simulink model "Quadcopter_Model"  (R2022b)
settings: Solver=VariableStepAuto  StartTime=0.0  StopTime=runtime  FixedStep=0.001  RelTol=1e-3
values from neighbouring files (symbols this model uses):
  delta_T = [ 0,  0,  9.404e-04 ]    [modelParameters.m]    (also in rich_params.m = [ 0,  0,  1.176e-04 ]; drone_control_system_test.m)
  g = 9.81    [modelParameters.m]    (also in rich_params.m; drone_control_system_test.m; imu_model_test.m = 0.1)
  height_controlled_o = (((Rm*If        + (((omega0_o * 2 * Rm * Kv * Kq      * Kd + 1)^2) - 1)/(4* Rm*Kv^2*Kq      * Kd))/Vb)*(Pmax - Pmin) + Pmin)    [modelParameters.m]    (also in rich_params.m)
  If = 0.3836    [modelParameters.m]    (also in rich_params.m = 0.39; drone_control_system_test.m)
  Jreq = 4.2012e-05    [modelParameters.m]    (also in rich_params.m = 1.376e-05; drone_control_system_test.m)
  Jxx = 0.0110    (= 0.011)    [modelParameters.m]    (also in rich_params.m = 0.0081; drone_control_system_test.m)
  Jyy = 0.0116    [modelParameters.m]    (also in rich_params.m = 0.0074; drone_control_system_test.m)
  Jzz = 0.0223    [modelParameters.m]    (also in rich_params.m = 0.0135; drone_control_system_test.m)
  Kd = 1.4852e-07    [modelParameters.m]    (also in rich_params.m = 5.194e-07; drone_control_system_test.m)
  Kh = 3.4574e-04    (= 0.00034574)    [modelParameters.m]    (also in rich_params.m; drone_control_system_test.m)
  Kq = 96.3422    [modelParameters.m]    (also in rich_params.m = 110; drone_control_system_test.m)
  Kt = 1.2007e-05    [modelParameters.m]    (also in rich_params.m = 7.3956e-06; drone_control_system_test.m)
  Kv = 96.3422    [modelParameters.m]    (also in rich_params.m = 110; drone_control_system_test.m)
  m = 1.216    [modelParameters.m]    (also in rich_params.m = 0.656; drone_control_system_test.m)
  omega0_o = sqrt((m*g)/(4*Kt))    [modelParameters.m]    (also in rich_params.m)
  omega1_o = sqrt((m*g)/(4*Kt))    [modelParameters.m]    (also in rich_params.m)
  omega2_o = sqrt((m*g)/(4*Kt))    [modelParameters.m]    (also in rich_params.m)
  omega3_o = sqrt((m*g)/(4*Kt))    [modelParameters.m]    (also in rich_params.m)
  pitch_o = 0    [modelParameters.m]    (also in rich_params.m)
  pitchrate_o = 0    [modelParameters.m]    (also in rich_params.m)
  Pmax = 1    [modelParameters.m]    (also in rich_params.m; drone_control_system_test.m)
  Pmin = 0    [modelParameters.m]    (also in rich_params.m; drone_control_system_test.m)
  r_oc = [ 0 ; 0 ; 0 ]    [modelParameters.m]    (also in rich_params.m; drone_control_system_test.m = [0; 0; 0]; imu_model_test.m = 0.1)
  rhx = 0.16    [modelParameters.m]    (also in rich_params.m = 0.115; drone_control_system_test.m)
  rhy = 0.16    [modelParameters.m]    (also in rich_params.m = 0.115; drone_control_system_test.m)
  rhz = 0.03    [modelParameters.m]    (also in rich_params.m = 0.04; drone_control_system_test.m)
  Rm = 0.235    [modelParameters.m]    (also in rich_params.m = 0.19; drone_control_system_test.m)
  roll_o = 0    [modelParameters.m]    (also in rich_params.m)
  rollrate_o = 0    [modelParameters.m]    (also in rich_params.m)
  signal_mixer = [ 1, -1, -1, -1    [modelParameters.m]    (also in rich_params.m; drone_control_system_test.m)
  Tc = 0.01    [modelParameters.m]    (also in rich_params.m; drone_control_system_test.m)
  Tq = 0.005    [modelParameters.m]    (also in rich_params.m; drone_control_system_test.m)
  Vb = 12.3    [modelParameters.m]    (also in rich_params.m = 11.4; drone_control_system_test.m)
  x_controlled_o = 0    [modelParameters.m]    (also in rich_params.m)
  x_o = 0    [modelParameters.m]    (also in rich_params.m)
  x_vel_o = 0    [modelParameters.m]    (also in rich_params.m)
  y_controlled_o = 0    [modelParameters.m]    (also in rich_params.m)
  y_o = 0    [modelParameters.m]    (also in rich_params.m)
  y_vel_o = 0    [modelParameters.m]    (also in rich_params.m)
  yaw_controlled_o = 0    [modelParameters.m]    (also in rich_params.m)
  yaw_o = 0    [modelParameters.m]    (also in rich_params.m)
  yawrate_o = 0    [modelParameters.m]    (also in rich_params.m)
  z_o = 0    [modelParameters.m]    (also in rich_params.m)
  z_vel_o = 0    [modelParameters.m]    (also in rich_params.m)
undefined symbols (not defined in the file or in its folder): lqr_K
libraries: Derivative x13, slpidlib x13, dsparch4 x3, vrlib x2, simulink_need_slupdate x2, simulink x1
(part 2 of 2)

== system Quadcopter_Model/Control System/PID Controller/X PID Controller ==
  x_error : Inport
  x_pos : Inport  Port=2
  Add : Sum  Inputs=+-
  Discrete D Controller : Derivative/Discrete D Controller  Kd=Kd  a=a
  Discrete PI Controller : slpidlib/PID Controller  Controller=PI  Form=Parallel  TimeDomain=Discrete-time  UseExternalTs=off  SampleTime=Ts  IntegratorMethod=Forward Euler  FilterMethod=Forward Euler  ControllerParametersSource=internal  P=Kp  I=Ki  UseKiTs=off  D=0  N=100  UseFilter=on  TunerSelectOption=Transfer Function Based (PID Tuner App)  InitialConditionSource=internal  InitialConditionForIntegrator=0  InitialConditionForFilter=0  DifferentiatorICPrevScaledInput=0  ExternalReset=none  TrackingMode=off  Kt=1  LimitOutput=off  SatLimitsSource=internal  UpperSaturationLimit=inf  LowerSaturationLimit=-inf  LinearizeAsGain=off  AntiWindupMode=none  Kb=1  LimitIntegrator=off  UpperIntegratorSaturationLimit=inf  LowerIntegratorSaturationLimit=-inf  POutMin=[]  POutMax=[]  IOutMin=[]  IOutMax=[]  DOutMin=[]  DOutMax=[]  NOutMin=[]  NOutMax=[]  SumOutMin=[]  SumOutMax=[]  SaturationOutMin=[]  SaturationOutMax=[]  PParamMin=[]  PParamMax=[]  IParamMin=[]  IParamMax=[]  DParamMin=[]  DParamMax=[]  NParamMin=[]  NParamMax=[]  KbParamMin=[]  KbParamMax=[]  KtParamMin=[]  KtParamMax=[]  KbOutMin=[]  KbOutMax=[]  KtOutMin=[]  KtOutMax=[]  IntegratorOutMin=[]  IntegratorOutMax=[]  FilterOutMin=[]  FilterOutMax=[]  SumI1OutMin=[]  SumI1OutMax=[]  SumI2OutMin=[]  SumI2OutMax=[]  SumI3OutMin=[]  SumI3OutMax=[]  SumI4OutMin=[]  SumI4OutMax=[]  SumDOutMin=[]  SumDOutMax=[]  DifferentiatorOutMin=[]  DifferentiatorOutMax=[]  FilterDiffOutCoefMin=[]  FilterDiffOutCoefMax=[]  ReciprocalOutMin=[]  ReciprocalOutMax=[]  SumDenOutMin=[]  SumDenOutMax=[]  SumNumOutMin=[]  SumNumOutMax=[]  DivideOutMin=[]  DivideOutMax=[]  UdiffTsProdOutMin=[]  UdiffTsProdOutMax=[]  NTsProdOutMin=[]  NTsProdOutMax=[]  UintegralTsProdOutMin=[]  UintegralTsProdOutMax=[]  UngainTsProdOutMin=[]  UngainTsProdOutMax=[]  ClampingZeroOutDataTypeStr=Inherit: Inherit via back propagation  ClampingZeroOutMin=[]  ClampingZeroOutMax=[]  FilterDenConstantOutDataTypeStr=Inherit: Inherit via back propagation  FilterDenConstantOutMin=[]  FilterDenConstantOutMax=[]  PCopyOutDataTypeStr=Inherit: Inherit via back propagation  PCopyOutMin=[]  PCopyOutMax=[]  NCopyOutDataTypeStr=Inherit: Inherit via back propagation  NCopyOutMin=[]  NCopyOutMax=[]  IntegratorContinuousStateAttributes=''  IntegratorStateMustResolveToSignalObject=off  IntegratorRTWStateStorageClass=Auto  FilterContinuousStateAttributes=''  FilterStateMustResolveToSignalObject=off  FilterRTWStateStorageClass=Auto  ParallelPVariant=InternalParameters  IdealPVariant=Disabled  IVariant=InternalParameters  DVariant=Disabled  IntegratorVariant=Discrete  SatVariant=Disabled  AWVariant=Passthrough  PCopyVariant=Disabled  TRVariant=Disabled  FdbkBlocksVariant=Forward  IdealPFdbkVariant=Disabled  SatFdbkVariant=Disabled  DerivativeFilterVariant=Disabled  NVariant=Disabled  NCopyVariant=Disabled_SignalSpec  FilterICVariant=Disabled  IntegratorICVariant=InternalICs  ExternalResetVariant=Disabled  TRSumVariant=Passthrough  SumFdbkVariant=Disabled  SumVariant=Sum_PI  TsampFilterVariant=InternalTs  TsampNgainVariant=Passthrough  TsampIntegralVariant=Passthrough  ExternalSaturationOutDataTypeStr=Inherit: Same as second input
  pitch_setpoint : Outport
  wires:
  x_pos/1 -> Discrete D Controller/1
  x_error/1 -> Discrete PI Controller/1
  Discrete PI Controller/1 -> Add/1
  Discrete D Controller/1 -> Add/2
  Add/1 -> pitch_setpoint/1

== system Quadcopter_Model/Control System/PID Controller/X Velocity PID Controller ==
  x_vel_error : Inport
  x_vel : Inport  Port=2
  Add : Sum  Inputs=+-
  Discrete D Controller : Derivative/Discrete D Controller  Kd=Kd  a=a
  Discrete PI Controller : slpidlib/PID Controller  Controller=PI  Form=Parallel  TimeDomain=Discrete-time  UseExternalTs=off  SampleTime=Ts  IntegratorMethod=Forward Euler  FilterMethod=Forward Euler  ControllerParametersSource=internal  P=Kp  I=Ki  UseKiTs=off  D=0  N=100  UseFilter=on  TunerSelectOption=Transfer Function Based (PID Tuner App)  InitialConditionSource=internal  InitialConditionForIntegrator=0  InitialConditionForFilter=0  DifferentiatorICPrevScaledInput=0  ExternalReset=none  TrackingMode=off  Kt=1  LimitOutput=off  SatLimitsSource=internal  UpperSaturationLimit=inf  LowerSaturationLimit=-inf  LinearizeAsGain=off  AntiWindupMode=none  Kb=1  LimitIntegrator=off  UpperIntegratorSaturationLimit=inf  LowerIntegratorSaturationLimit=-inf  POutMin=[]  POutMax=[]  IOutMin=[]  IOutMax=[]  DOutMin=[]  DOutMax=[]  NOutMin=[]  NOutMax=[]  SumOutMin=[]  SumOutMax=[]  SaturationOutMin=[]  SaturationOutMax=[]  PParamMin=[]  PParamMax=[]  IParamMin=[]  IParamMax=[]  DParamMin=[]  DParamMax=[]  NParamMin=[]  NParamMax=[]  KbParamMin=[]  KbParamMax=[]  KtParamMin=[]  KtParamMax=[]  KbOutMin=[]  KbOutMax=[]  KtOutMin=[]  KtOutMax=[]  IntegratorOutMin=[]  IntegratorOutMax=[]  FilterOutMin=[]  FilterOutMax=[]  SumI1OutMin=[]  SumI1OutMax=[]  SumI2OutMin=[]  SumI2OutMax=[]  SumI3OutMin=[]  SumI3OutMax=[]  SumI4OutMin=[]  SumI4OutMax=[]  SumDOutMin=[]  SumDOutMax=[]  DifferentiatorOutMin=[]  DifferentiatorOutMax=[]  FilterDiffOutCoefMin=[]  FilterDiffOutCoefMax=[]  ReciprocalOutMin=[]  ReciprocalOutMax=[]  SumDenOutMin=[]  SumDenOutMax=[]  SumNumOutMin=[]  SumNumOutMax=[]  DivideOutMin=[]  DivideOutMax=[]  UdiffTsProdOutMin=[]  UdiffTsProdOutMax=[]  NTsProdOutMin=[]  NTsProdOutMax=[]  UintegralTsProdOutMin=[]  UintegralTsProdOutMax=[]  UngainTsProdOutMin=[]  UngainTsProdOutMax=[]  ClampingZeroOutDataTypeStr=Inherit: Inherit via back propagation  ClampingZeroOutMin=[]  ClampingZeroOutMax=[]  FilterDenConstantOutDataTypeStr=Inherit: Inherit via back propagation  FilterDenConstantOutMin=[]  FilterDenConstantOutMax=[]  PCopyOutDataTypeStr=Inherit: Inherit via back propagation  PCopyOutMin=[]  PCopyOutMax=[]  NCopyOutDataTypeStr=Inherit: Inherit via back propagation  NCopyOutMin=[]  NCopyOutMax=[]  IntegratorContinuousStateAttributes=''  IntegratorStateMustResolveToSignalObject=off  IntegratorRTWStateStorageClass=Auto  FilterContinuousStateAttributes=''  FilterStateMustResolveToSignalObject=off  FilterRTWStateStorageClass=Auto  ParallelPVariant=InternalParameters  IdealPVariant=Disabled  IVariant=InternalParameters  DVariant=Disabled  IntegratorVariant=Discrete  SatVariant=Disabled  AWVariant=Passthrough  PCopyVariant=Disabled  TRVariant=Disabled  FdbkBlocksVariant=Forward  IdealPFdbkVariant=Disabled  SatFdbkVariant=Disabled  DerivativeFilterVariant=Disabled  NVariant=Disabled  NCopyVariant=Disabled_SignalSpec  FilterICVariant=Disabled  IntegratorICVariant=InternalICs  ExternalResetVariant=Disabled  TRSumVariant=Passthrough  SumFdbkVariant=Disabled  SumVariant=Sum_PI  TsampFilterVariant=InternalTs  TsampNgainVariant=Passthrough  TsampIntegralVariant=Passthrough  ExternalSaturationOutDataTypeStr=Inherit: Same as second input
  pitch_setpoint : Outport
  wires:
  x_vel/1 -> Discrete D Controller/1
  x_vel_error/1 -> Discrete PI Controller/1
  Discrete PI Controller/1 -> Add/1
  Discrete D Controller/1 -> Add/2
  Add/1 -> pitch_setpoint/1

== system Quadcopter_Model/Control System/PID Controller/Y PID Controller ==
  y_error : Inport
  y_pos : Inport  Port=2
  Add : Sum  Inputs=+-
  Discrete D Controller : Derivative/Discrete D Controller  Kd=Kd  a=a
  Discrete PI Controller : slpidlib/PID Controller  Controller=PI  Form=Parallel  TimeDomain=Discrete-time  UseExternalTs=off  SampleTime=Ts  IntegratorMethod=Forward Euler  FilterMethod=Forward Euler  ControllerParametersSource=internal  P=Kp  I=Ki  UseKiTs=off  D=0  N=100  UseFilter=on  TunerSelectOption=Transfer Function Based (PID Tuner App)  InitialConditionSource=internal  InitialConditionForIntegrator=0  InitialConditionForFilter=0  DifferentiatorICPrevScaledInput=0  ExternalReset=none  TrackingMode=off  Kt=1  LimitOutput=off  SatLimitsSource=internal  UpperSaturationLimit=inf  LowerSaturationLimit=-inf  LinearizeAsGain=off  AntiWindupMode=none  Kb=1  LimitIntegrator=off  UpperIntegratorSaturationLimit=inf  LowerIntegratorSaturationLimit=-inf  POutMin=[]  POutMax=[]  IOutMin=[]  IOutMax=[]  DOutMin=[]  DOutMax=[]  NOutMin=[]  NOutMax=[]  SumOutMin=[]  SumOutMax=[]  SaturationOutMin=[]  SaturationOutMax=[]  PParamMin=[]  PParamMax=[]  IParamMin=[]  IParamMax=[]  DParamMin=[]  DParamMax=[]  NParamMin=[]  NParamMax=[]  KbParamMin=[]  KbParamMax=[]  KtParamMin=[]  KtParamMax=[]  KbOutMin=[]  KbOutMax=[]  KtOutMin=[]  KtOutMax=[]  IntegratorOutMin=[]  IntegratorOutMax=[]  FilterOutMin=[]  FilterOutMax=[]  SumI1OutMin=[]  SumI1OutMax=[]  SumI2OutMin=[]  SumI2OutMax=[]  SumI3OutMin=[]  SumI3OutMax=[]  SumI4OutMin=[]  SumI4OutMax=[]  SumDOutMin=[]  SumDOutMax=[]  DifferentiatorOutMin=[]  DifferentiatorOutMax=[]  FilterDiffOutCoefMin=[]  FilterDiffOutCoefMax=[]  ReciprocalOutMin=[]  ReciprocalOutMax=[]  SumDenOutMin=[]  SumDenOutMax=[]  SumNumOutMin=[]  SumNumOutMax=[]  DivideOutMin=[]  DivideOutMax=[]  UdiffTsProdOutMin=[]  UdiffTsProdOutMax=[]  NTsProdOutMin=[]  NTsProdOutMax=[]  UintegralTsProdOutMin=[]  UintegralTsProdOutMax=[]  UngainTsProdOutMin=[]  UngainTsProdOutMax=[]  ClampingZeroOutDataTypeStr=Inherit: Inherit via back propagation  ClampingZeroOutMin=[]  ClampingZeroOutMax=[]  FilterDenConstantOutDataTypeStr=Inherit: Inherit via back propagation  FilterDenConstantOutMin=[]  FilterDenConstantOutMax=[]  PCopyOutDataTypeStr=Inherit: Inherit via back propagation  PCopyOutMin=[]  PCopyOutMax=[]  NCopyOutDataTypeStr=Inherit: Inherit via back propagation  NCopyOutMin=[]  NCopyOutMax=[]  IntegratorContinuousStateAttributes=''  IntegratorStateMustResolveToSignalObject=off  IntegratorRTWStateStorageClass=Auto  FilterContinuousStateAttributes=''  FilterStateMustResolveToSignalObject=off  FilterRTWStateStorageClass=Auto  ParallelPVariant=InternalParameters  IdealPVariant=Disabled  IVariant=InternalParameters  DVariant=Disabled  IntegratorVariant=Discrete  SatVariant=Disabled  AWVariant=Passthrough  PCopyVariant=Disabled  TRVariant=Disabled  FdbkBlocksVariant=Forward  IdealPFdbkVariant=Disabled  SatFdbkVariant=Disabled  DerivativeFilterVariant=Disabled  NVariant=Disabled  NCopyVariant=Disabled_SignalSpec  FilterICVariant=Disabled  IntegratorICVariant=InternalICs  ExternalResetVariant=Disabled  TRSumVariant=Passthrough  SumFdbkVariant=Disabled  SumVariant=Sum_PI  TsampFilterVariant=InternalTs  TsampNgainVariant=Passthrough  TsampIntegralVariant=Passthrough  ExternalSaturationOutDataTypeStr=Inherit: Same as second input
  roll_setpoint : Outport
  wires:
  y_pos/1 -> Discrete D Controller/1
  y_error/1 -> Discrete PI Controller/1
  Discrete PI Controller/1 -> Add/1
  Discrete D Controller/1 -> Add/2
  Add/1 -> roll_setpoint/1

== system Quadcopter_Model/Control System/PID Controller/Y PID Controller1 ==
  y_error : Inport
  y_pos : Inport  Port=2
  Add : Sum  Inputs=+-
  Discrete D Controller : Derivative/Discrete D Controller  Kd=Kd  a=a
  Discrete PI Controller : slpidlib/PID Controller  Controller=PI  Form=Parallel  TimeDomain=Discrete-time  UseExternalTs=off  SampleTime=Ts  IntegratorMethod=Forward Euler  FilterMethod=Forward Euler  ControllerParametersSource=internal  P=Kp  I=Ki  UseKiTs=off  D=0  N=100  UseFilter=on  TunerSelectOption=Transfer Function Based (PID Tuner App)  InitialConditionSource=internal  InitialConditionForIntegrator=0  InitialConditionForFilter=0  DifferentiatorICPrevScaledInput=0  ExternalReset=none  TrackingMode=off  Kt=1  LimitOutput=off  SatLimitsSource=internal  UpperSaturationLimit=inf  LowerSaturationLimit=-inf  LinearizeAsGain=off  AntiWindupMode=none  Kb=1  LimitIntegrator=off  UpperIntegratorSaturationLimit=inf  LowerIntegratorSaturationLimit=-inf  POutMin=[]  POutMax=[]  IOutMin=[]  IOutMax=[]  DOutMin=[]  DOutMax=[]  NOutMin=[]  NOutMax=[]  SumOutMin=[]  SumOutMax=[]  SaturationOutMin=[]  SaturationOutMax=[]  PParamMin=[]  PParamMax=[]  IParamMin=[]  IParamMax=[]  DParamMin=[]  DParamMax=[]  NParamMin=[]  NParamMax=[]  KbParamMin=[]  KbParamMax=[]  KtParamMin=[]  KtParamMax=[]  KbOutMin=[]  KbOutMax=[]  KtOutMin=[]  KtOutMax=[]  IntegratorOutMin=[]  IntegratorOutMax=[]  FilterOutMin=[]  FilterOutMax=[]  SumI1OutMin=[]  SumI1OutMax=[]  SumI2OutMin=[]  SumI2OutMax=[]  SumI3OutMin=[]  SumI3OutMax=[]  SumI4OutMin=[]  SumI4OutMax=[]  SumDOutMin=[]  SumDOutMax=[]  DifferentiatorOutMin=[]  DifferentiatorOutMax=[]  FilterDiffOutCoefMin=[]  FilterDiffOutCoefMax=[]  ReciprocalOutMin=[]  ReciprocalOutMax=[]  SumDenOutMin=[]  SumDenOutMax=[]  SumNumOutMin=[]  SumNumOutMax=[]  DivideOutMin=[]  DivideOutMax=[]  UdiffTsProdOutMin=[]  UdiffTsProdOutMax=[]  NTsProdOutMin=[]  NTsProdOutMax=[]  UintegralTsProdOutMin=[]  UintegralTsProdOutMax=[]  UngainTsProdOutMin=[]  UngainTsProdOutMax=[]  ClampingZeroOutDataTypeStr=Inherit: Inherit via back propagation  ClampingZeroOutMin=[]  ClampingZeroOutMax=[]  FilterDenConstantOutDataTypeStr=Inherit: Inherit via back propagation  FilterDenConstantOutMin=[]  FilterDenConstantOutMax=[]  PCopyOutDataTypeStr=Inherit: Inherit via back propagation  PCopyOutMin=[]  PCopyOutMax=[]  NCopyOutDataTypeStr=Inherit: Inherit via back propagation  NCopyOutMin=[]  NCopyOutMax=[]  IntegratorContinuousStateAttributes=''  IntegratorStateMustResolveToSignalObject=off  IntegratorRTWStateStorageClass=Auto  FilterContinuousStateAttributes=''  FilterStateMustResolveToSignalObject=off  FilterRTWStateStorageClass=Auto  ParallelPVariant=InternalParameters  IdealPVariant=Disabled  IVariant=InternalParameters  DVariant=Disabled  IntegratorVariant=Discrete  SatVariant=Disabled  AWVariant=Passthrough  PCopyVariant=Disabled  TRVariant=Disabled  FdbkBlocksVariant=Forward  IdealPFdbkVariant=Disabled  SatFdbkVariant=Disabled  DerivativeFilterVariant=Disabled  NVariant=Disabled  NCopyVariant=Disabled_SignalSpec  FilterICVariant=Disabled  IntegratorICVariant=InternalICs  ExternalResetVariant=Disabled  TRSumVariant=Passthrough  SumFdbkVariant=Disabled  SumVariant=Sum_PI  TsampFilterVariant=InternalTs  TsampNgainVariant=Passthrough  TsampIntegralVariant=Passthrough  ExternalSaturationOutDataTypeStr=Inherit: Same as second input
  y_vel_setpoint : Outport
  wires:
  y_pos/1 -> Discrete D Controller/1
  y_error/1 -> Discrete PI Controller/1
  Discrete PI Controller/1 -> Add/1
  Discrete D Controller/1 -> Add/2
  Add/1 -> y_vel_setpoint/1

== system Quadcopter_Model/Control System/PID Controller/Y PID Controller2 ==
  x_error : Inport
  x_pos : Inport  Port=2
  Add : Sum  Inputs=+-
  Discrete D Controller : Derivative/Discrete D Controller  Kd=Kd  a=a
  Discrete PI Controller : slpidlib/PID Controller  Controller=PI  Form=Parallel  TimeDomain=Discrete-time  UseExternalTs=off  SampleTime=Ts  IntegratorMethod=Forward Euler  FilterMethod=Forward Euler  ControllerParametersSource=internal  P=Kp  I=Ki  UseKiTs=off  D=0  N=100  UseFilter=on  TunerSelectOption=Transfer Function Based (PID Tuner App)  InitialConditionSource=internal  InitialConditionForIntegrator=0  InitialConditionForFilter=0  DifferentiatorICPrevScaledInput=0  ExternalReset=none  TrackingMode=off  Kt=1  LimitOutput=off  SatLimitsSource=internal  UpperSaturationLimit=inf  LowerSaturationLimit=-inf  LinearizeAsGain=off  AntiWindupMode=none  Kb=1  LimitIntegrator=off  UpperIntegratorSaturationLimit=inf  LowerIntegratorSaturationLimit=-inf  POutMin=[]  POutMax=[]  IOutMin=[]  IOutMax=[]  DOutMin=[]  DOutMax=[]  NOutMin=[]  NOutMax=[]  SumOutMin=[]  SumOutMax=[]  SaturationOutMin=[]  SaturationOutMax=[]  PParamMin=[]  PParamMax=[]  IParamMin=[]  IParamMax=[]  DParamMin=[]  DParamMax=[]  NParamMin=[]  NParamMax=[]  KbParamMin=[]  KbParamMax=[]  KtParamMin=[]  KtParamMax=[]  KbOutMin=[]  KbOutMax=[]  KtOutMin=[]  KtOutMax=[]  IntegratorOutMin=[]  IntegratorOutMax=[]  FilterOutMin=[]  FilterOutMax=[]  SumI1OutMin=[]  SumI1OutMax=[]  SumI2OutMin=[]  SumI2OutMax=[]  SumI3OutMin=[]  SumI3OutMax=[]  SumI4OutMin=[]  SumI4OutMax=[]  SumDOutMin=[]  SumDOutMax=[]  DifferentiatorOutMin=[]  DifferentiatorOutMax=[]  FilterDiffOutCoefMin=[]  FilterDiffOutCoefMax=[]  ReciprocalOutMin=[]  ReciprocalOutMax=[]  SumDenOutMin=[]  SumDenOutMax=[]  SumNumOutMin=[]  SumNumOutMax=[]  DivideOutMin=[]  DivideOutMax=[]  UdiffTsProdOutMin=[]  UdiffTsProdOutMax=[]  NTsProdOutMin=[]  NTsProdOutMax=[]  UintegralTsProdOutMin=[]  UintegralTsProdOutMax=[]  UngainTsProdOutMin=[]  UngainTsProdOutMax=[]  ClampingZeroOutDataTypeStr=Inherit: Inherit via back propagation  ClampingZeroOutMin=[]  ClampingZeroOutMax=[]  FilterDenConstantOutDataTypeStr=Inherit: Inherit via back propagation  FilterDenConstantOutMin=[]  FilterDenConstantOutMax=[]  PCopyOutDataTypeStr=Inherit: Inherit via back propagation  PCopyOutMin=[]  PCopyOutMax=[]  NCopyOutDataTypeStr=Inherit: Inherit via back propagation  NCopyOutMin=[]  NCopyOutMax=[]  IntegratorContinuousStateAttributes=''  IntegratorStateMustResolveToSignalObject=off  IntegratorRTWStateStorageClass=Auto  FilterContinuousStateAttributes=''  FilterStateMustResolveToSignalObject=off  FilterRTWStateStorageClass=Auto  ParallelPVariant=InternalParameters  IdealPVariant=Disabled  IVariant=InternalParameters  DVariant=Disabled  IntegratorVariant=Discrete  SatVariant=Disabled  AWVariant=Passthrough  PCopyVariant=Disabled  TRVariant=Disabled  FdbkBlocksVariant=Forward  IdealPFdbkVariant=Disabled  SatFdbkVariant=Disabled  DerivativeFilterVariant=Disabled  NVariant=Disabled  NCopyVariant=Disabled_SignalSpec  FilterICVariant=Disabled  IntegratorICVariant=InternalICs  ExternalResetVariant=Disabled  TRSumVariant=Passthrough  SumFdbkVariant=Disabled  SumVariant=Sum_PI  TsampFilterVariant=InternalTs  TsampNgainVariant=Passthrough  TsampIntegralVariant=Passthrough  ExternalSaturationOutDataTypeStr=Inherit: Same as second input
  x_vel_setpoint : Outport
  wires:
  x_pos/1 -> Discrete D Controller/1
  x_error/1 -> Discrete PI Controller/1
  Discrete PI Controller/1 -> Add/1
  Discrete D Controller/1 -> Add/2
  Add/1 -> x_vel_setpoint/1

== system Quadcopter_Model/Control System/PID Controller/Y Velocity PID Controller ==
  y_error : Inport
  y_pos : Inport  Port=2
  Add : Sum  Inputs=+-
  Discrete D Controller : Derivative/Discrete D Controller  Kd=Kd  a=a
  Discrete PI Controller : slpidlib/PID Controller  Controller=PI  Form=Parallel  TimeDomain=Discrete-time  UseExternalTs=off  SampleTime=Ts  IntegratorMethod=Forward Euler  FilterMethod=Forward Euler  ControllerParametersSource=internal  P=Kp  I=Ki  UseKiTs=off  D=0  N=100  UseFilter=on  TunerSelectOption=Transfer Function Based (PID Tuner App)  InitialConditionSource=internal  InitialConditionForIntegrator=0  InitialConditionForFilter=0  DifferentiatorICPrevScaledInput=0  ExternalReset=none  TrackingMode=off  Kt=1  LimitOutput=off  SatLimitsSource=internal  UpperSaturationLimit=inf  LowerSaturationLimit=-inf  LinearizeAsGain=off  AntiWindupMode=none  Kb=1  LimitIntegrator=off  UpperIntegratorSaturationLimit=inf  LowerIntegratorSaturationLimit=-inf  POutMin=[]  POutMax=[]  IOutMin=[]  IOutMax=[]  DOutMin=[]  DOutMax=[]  NOutMin=[]  NOutMax=[]  SumOutMin=[]  SumOutMax=[]  SaturationOutMin=[]  SaturationOutMax=[]  PParamMin=[]  PParamMax=[]  IParamMin=[]  IParamMax=[]  DParamMin=[]  DParamMax=[]  NParamMin=[]  NParamMax=[]  KbParamMin=[]  KbParamMax=[]  KtParamMin=[]  KtParamMax=[]  KbOutMin=[]  KbOutMax=[]  KtOutMin=[]  KtOutMax=[]  IntegratorOutMin=[]  IntegratorOutMax=[]  FilterOutMin=[]  FilterOutMax=[]  SumI1OutMin=[]  SumI1OutMax=[]  SumI2OutMin=[]  SumI2OutMax=[]  SumI3OutMin=[]  SumI3OutMax=[]  SumI4OutMin=[]  SumI4OutMax=[]  SumDOutMin=[]  SumDOutMax=[]  DifferentiatorOutMin=[]  DifferentiatorOutMax=[]  FilterDiffOutCoefMin=[]  FilterDiffOutCoefMax=[]  ReciprocalOutMin=[]  ReciprocalOutMax=[]  SumDenOutMin=[]  SumDenOutMax=[]  SumNumOutMin=[]  SumNumOutMax=[]  DivideOutMin=[]  DivideOutMax=[]  UdiffTsProdOutMin=[]  UdiffTsProdOutMax=[]  NTsProdOutMin=[]  NTsProdOutMax=[]  UintegralTsProdOutMin=[]  UintegralTsProdOutMax=[]  UngainTsProdOutMin=[]  UngainTsProdOutMax=[]  ClampingZeroOutDataTypeStr=Inherit: Inherit via back propagation  ClampingZeroOutMin=[]  ClampingZeroOutMax=[]  FilterDenConstantOutDataTypeStr=Inherit: Inherit via back propagation  FilterDenConstantOutMin=[]  FilterDenConstantOutMax=[]  PCopyOutDataTypeStr=Inherit: Inherit via back propagation  PCopyOutMin=[]  PCopyOutMax=[]  NCopyOutDataTypeStr=Inherit: Inherit via back propagation  NCopyOutMin=[]  NCopyOutMax=[]  IntegratorContinuousStateAttributes=''  IntegratorStateMustResolveToSignalObject=off  IntegratorRTWStateStorageClass=Auto  FilterContinuousStateAttributes=''  FilterStateMustResolveToSignalObject=off  FilterRTWStateStorageClass=Auto  ParallelPVariant=InternalParameters  IdealPVariant=Disabled  IVariant=InternalParameters  DVariant=Disabled  IntegratorVariant=Discrete  SatVariant=Disabled  AWVariant=Passthrough  PCopyVariant=Disabled  TRVariant=Disabled  FdbkBlocksVariant=Forward  IdealPFdbkVariant=Disabled  SatFdbkVariant=Disabled  DerivativeFilterVariant=Disabled  NVariant=Disabled  NCopyVariant=Disabled_SignalSpec  FilterICVariant=Disabled  IntegratorICVariant=InternalICs  ExternalResetVariant=Disabled  TRSumVariant=Passthrough  SumFdbkVariant=Disabled  SumVariant=Sum_PI  TsampFilterVariant=InternalTs  TsampNgainVariant=Passthrough  TsampIntegralVariant=Passthrough  ExternalSaturationOutDataTypeStr=Inherit: Same as second input
  roll_setpoint : Outport
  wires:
  y_pos/1 -> Discrete D Controller/1
  y_error/1 -> Discrete PI Controller/1
  Discrete PI Controller/1 -> Add/1
  Discrete D Controller/1 -> Add/2
  Add/1 -> roll_setpoint/1

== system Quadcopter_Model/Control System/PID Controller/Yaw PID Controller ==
  yaw_error : Inport
  yaw_angle : Inport  Port=2
  Add : Sum  Inputs=+-
  Discrete D Controller : Derivative/Discrete D Controller  Kd=Kd  a=a
  Discrete PI Controller : slpidlib/PID Controller  Controller=PI  Form=Parallel  TimeDomain=Discrete-time  UseExternalTs=off  SampleTime=Ts  IntegratorMethod=Forward Euler  FilterMethod=Forward Euler  ControllerParametersSource=internal  P=Kp  I=Ki  UseKiTs=off  D=0  N=100  UseFilter=on  TunerSelectOption=Transfer Function Based (PID Tuner App)  InitialConditionSource=internal  InitialConditionForIntegrator=0  InitialConditionForFilter=0  DifferentiatorICPrevScaledInput=0  ExternalReset=none  TrackingMode=off  Kt=1  LimitOutput=off  SatLimitsSource=internal  UpperSaturationLimit=inf  LowerSaturationLimit=-inf  LinearizeAsGain=off  AntiWindupMode=none  Kb=1  LimitIntegrator=off  UpperIntegratorSaturationLimit=inf  LowerIntegratorSaturationLimit=-inf  POutMin=[]  POutMax=[]  IOutMin=[]  IOutMax=[]  DOutMin=[]  DOutMax=[]  NOutMin=[]  NOutMax=[]  SumOutMin=[]  SumOutMax=[]  SaturationOutMin=[]  SaturationOutMax=[]  PParamMin=[]  PParamMax=[]  IParamMin=[]  IParamMax=[]  DParamMin=[]  DParamMax=[]  NParamMin=[]  NParamMax=[]  KbParamMin=[]  KbParamMax=[]  KtParamMin=[]  KtParamMax=[]  KbOutMin=[]  KbOutMax=[]  KtOutMin=[]  KtOutMax=[]  IntegratorOutMin=[]  IntegratorOutMax=[]  FilterOutMin=[]  FilterOutMax=[]  SumI1OutMin=[]  SumI1OutMax=[]  SumI2OutMin=[]  SumI2OutMax=[]  SumI3OutMin=[]  SumI3OutMax=[]  SumI4OutMin=[]  SumI4OutMax=[]  SumDOutMin=[]  SumDOutMax=[]  DifferentiatorOutMin=[]  DifferentiatorOutMax=[]  FilterDiffOutCoefMin=[]  FilterDiffOutCoefMax=[]  ReciprocalOutMin=[]  ReciprocalOutMax=[]  SumDenOutMin=[]  SumDenOutMax=[]  SumNumOutMin=[]  SumNumOutMax=[]  DivideOutMin=[]  DivideOutMax=[]  UdiffTsProdOutMin=[]  UdiffTsProdOutMax=[]  NTsProdOutMin=[]  NTsProdOutMax=[]  UintegralTsProdOutMin=[]  UintegralTsProdOutMax=[]  UngainTsProdOutMin=[]  UngainTsProdOutMax=[]  ClampingZeroOutDataTypeStr=Inherit: Inherit via back propagation  ClampingZeroOutMin=[]  ClampingZeroOutMax=[]  FilterDenConstantOutDataTypeStr=Inherit: Inherit via back propagation  FilterDenConstantOutMin=[]  FilterDenConstantOutMax=[]  PCopyOutDataTypeStr=Inherit: Inherit via back propagation  PCopyOutMin=[]  PCopyOutMax=[]  NCopyOutDataTypeStr=Inherit: Inherit via back propagation  NCopyOutMin=[]  NCopyOutMax=[]  IntegratorContinuousStateAttributes=''  IntegratorStateMustResolveToSignalObject=off  IntegratorRTWStateStorageClass=Auto  FilterContinuousStateAttributes=''  FilterStateMustResolveToSignalObject=off  FilterRTWStateStorageClass=Auto  ParallelPVariant=InternalParameters  IdealPVariant=Disabled  IVariant=InternalParameters  DVariant=Disabled  IntegratorVariant=Discrete  SatVariant=Disabled  AWVariant=Passthrough  PCopyVariant=Disabled  TRVariant=Disabled  FdbkBlocksVariant=Forward  IdealPFdbkVariant=Disabled  SatFdbkVariant=Disabled  DerivativeFilterVariant=Disabled  NVariant=Disabled  NCopyVariant=Disabled_SignalSpec  FilterICVariant=Disabled  IntegratorICVariant=InternalICs  ExternalResetVariant=Disabled  TRSumVariant=Passthrough  SumFdbkVariant=Disabled  SumVariant=Sum_PI  TsampFilterVariant=InternalTs  TsampNgainVariant=Passthrough  TsampIntegralVariant=Passthrough  ExternalSaturationOutDataTypeStr=Inherit: Same as second input
  yawrate_setpoint : Outport
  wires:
  yaw_angle/1 -> Discrete D Controller/1
  yaw_error/1 -> Discrete PI Controller/1
  Discrete PI Controller/1 -> Add/1
  Discrete D Controller/1 -> Add/2
  Add/1 -> yawrate_setpoint/1

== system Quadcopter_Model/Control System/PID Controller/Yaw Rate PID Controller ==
  yawrate_error : Inport
  yawrate : Inport  Port=2
  Add : Sum  Inputs=+-
  Discrete D Controller : Derivative/Discrete D Controller  Kd=Kd  a=a
  Discrete PI Controller : slpidlib/PID Controller  Controller=PI  Form=Parallel  TimeDomain=Discrete-time  UseExternalTs=off  SampleTime=Ts  IntegratorMethod=Forward Euler  FilterMethod=Forward Euler  ControllerParametersSource=internal  P=Kp  I=Ki  UseKiTs=off  D=0  N=100  UseFilter=on  TunerSelectOption=Transfer Function Based (PID Tuner App)  InitialConditionSource=internal  InitialConditionForIntegrator=0  InitialConditionForFilter=0  DifferentiatorICPrevScaledInput=0  ExternalReset=none  TrackingMode=off  Kt=1  LimitOutput=off  SatLimitsSource=internal  UpperSaturationLimit=inf  LowerSaturationLimit=-inf  LinearizeAsGain=off  AntiWindupMode=none  Kb=1  LimitIntegrator=off  UpperIntegratorSaturationLimit=inf  LowerIntegratorSaturationLimit=-inf  POutMin=[]  POutMax=[]  IOutMin=[]  IOutMax=[]  DOutMin=[]  DOutMax=[]  NOutMin=[]  NOutMax=[]  SumOutMin=[]  SumOutMax=[]  SaturationOutMin=[]  SaturationOutMax=[]  PParamMin=[]  PParamMax=[]  IParamMin=[]  IParamMax=[]  DParamMin=[]  DParamMax=[]  NParamMin=[]  NParamMax=[]  KbParamMin=[]  KbParamMax=[]  KtParamMin=[]  KtParamMax=[]  KbOutMin=[]  KbOutMax=[]  KtOutMin=[]  KtOutMax=[]  IntegratorOutMin=[]  IntegratorOutMax=[]  FilterOutMin=[]  FilterOutMax=[]  SumI1OutMin=[]  SumI1OutMax=[]  SumI2OutMin=[]  SumI2OutMax=[]  SumI3OutMin=[]  SumI3OutMax=[]  SumI4OutMin=[]  SumI4OutMax=[]  SumDOutMin=[]  SumDOutMax=[]  DifferentiatorOutMin=[]  DifferentiatorOutMax=[]  FilterDiffOutCoefMin=[]  FilterDiffOutCoefMax=[]  ReciprocalOutMin=[]  ReciprocalOutMax=[]  SumDenOutMin=[]  SumDenOutMax=[]  SumNumOutMin=[]  SumNumOutMax=[]  DivideOutMin=[]  DivideOutMax=[]  UdiffTsProdOutMin=[]  UdiffTsProdOutMax=[]  NTsProdOutMin=[]  NTsProdOutMax=[]  UintegralTsProdOutMin=[]  UintegralTsProdOutMax=[]  UngainTsProdOutMin=[]  UngainTsProdOutMax=[]  ClampingZeroOutDataTypeStr=Inherit: Inherit via back propagation  ClampingZeroOutMin=[]  ClampingZeroOutMax=[]  FilterDenConstantOutDataTypeStr=Inherit: Inherit via back propagation  FilterDenConstantOutMin=[]  FilterDenConstantOutMax=[]  PCopyOutDataTypeStr=Inherit: Inherit via back propagation  PCopyOutMin=[]  PCopyOutMax=[]  NCopyOutDataTypeStr=Inherit: Inherit via back propagation  NCopyOutMin=[]  NCopyOutMax=[]  IntegratorContinuousStateAttributes=''  IntegratorStateMustResolveToSignalObject=off  IntegratorRTWStateStorageClass=Auto  FilterContinuousStateAttributes=''  FilterStateMustResolveToSignalObject=off  FilterRTWStateStorageClass=Auto  ParallelPVariant=InternalParameters  IdealPVariant=Disabled  IVariant=InternalParameters  DVariant=Disabled  IntegratorVariant=Discrete  SatVariant=Disabled  AWVariant=Passthrough  PCopyVariant=Disabled  TRVariant=Disabled  FdbkBlocksVariant=Forward  IdealPFdbkVariant=Disabled  SatFdbkVariant=Disabled  DerivativeFilterVariant=Disabled  NVariant=Disabled  NCopyVariant=Disabled_SignalSpec  FilterICVariant=Disabled  IntegratorICVariant=InternalICs  ExternalResetVariant=Disabled  TRSumVariant=Passthrough  SumFdbkVariant=Disabled  SumVariant=Sum_PI  TsampFilterVariant=InternalTs  TsampNgainVariant=Passthrough  TsampIntegralVariant=Passthrough  ExternalSaturationOutDataTypeStr=Inherit: Same as second input
  yaw_motor_command : Outport
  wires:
  yawrate/1 -> Discrete D Controller/1
  yawrate_error/1 -> Discrete PI Controller/1
  Discrete PI Controller/1 -> Add/1
  Discrete D Controller/1 -> Add/2
  Add/1 -> yaw_motor_command/1

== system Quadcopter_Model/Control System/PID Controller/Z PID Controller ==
  z_error : Inport
  z_pos : Inport  Port=2
  Add : Sum  Inputs=+-
  Discrete D Controller : Derivative/Discrete D Controller  Kd=Kd  a=a
  Discrete PI Controller : slpidlib/PID Controller  Controller=PI  Form=Parallel  TimeDomain=Discrete-time  UseExternalTs=off  SampleTime=Ts  IntegratorMethod=Forward Euler  FilterMethod=Forward Euler  ControllerParametersSource=internal  P=Kp  I=Ki  UseKiTs=off  D=0  N=100  UseFilter=on  TunerSelectOption=Transfer Function Based (PID Tuner App)  InitialConditionSource=internal  InitialConditionForIntegrator=0  InitialConditionForFilter=0  DifferentiatorICPrevScaledInput=0  ExternalReset=none  TrackingMode=off  Kt=1  LimitOutput=off  SatLimitsSource=internal  UpperSaturationLimit=inf  LowerSaturationLimit=-inf  LinearizeAsGain=off  AntiWindupMode=none  Kb=1  LimitIntegrator=off  UpperIntegratorSaturationLimit=inf  LowerIntegratorSaturationLimit=-inf  POutMin=[]  POutMax=[]  IOutMin=[]  IOutMax=[]  DOutMin=[]  DOutMax=[]  NOutMin=[]  NOutMax=[]  SumOutMin=[]  SumOutMax=[]  SaturationOutMin=[]  SaturationOutMax=[]  PParamMin=[]  PParamMax=[]  IParamMin=[]  IParamMax=[]  DParamMin=[]  DParamMax=[]  NParamMin=[]  NParamMax=[]  KbParamMin=[]  KbParamMax=[]  KtParamMin=[]  KtParamMax=[]  KbOutMin=[]  KbOutMax=[]  KtOutMin=[]  KtOutMax=[]  IntegratorOutMin=[]  IntegratorOutMax=[]  FilterOutMin=[]  FilterOutMax=[]  SumI1OutMin=[]  SumI1OutMax=[]  SumI2OutMin=[]  SumI2OutMax=[]  SumI3OutMin=[]  SumI3OutMax=[]  SumI4OutMin=[]  SumI4OutMax=[]  SumDOutMin=[]  SumDOutMax=[]  DifferentiatorOutMin=[]  DifferentiatorOutMax=[]  FilterDiffOutCoefMin=[]  FilterDiffOutCoefMax=[]  ReciprocalOutMin=[]  ReciprocalOutMax=[]  SumDenOutMin=[]  SumDenOutMax=[]  SumNumOutMin=[]  SumNumOutMax=[]  DivideOutMin=[]  DivideOutMax=[]  UdiffTsProdOutMin=[]  UdiffTsProdOutMax=[]  NTsProdOutMin=[]  NTsProdOutMax=[]  UintegralTsProdOutMin=[]  UintegralTsProdOutMax=[]  UngainTsProdOutMin=[]  UngainTsProdOutMax=[]  ClampingZeroOutDataTypeStr=Inherit: Inherit via back propagation  ClampingZeroOutMin=[]  ClampingZeroOutMax=[]  FilterDenConstantOutDataTypeStr=Inherit: Inherit via back propagation  FilterDenConstantOutMin=[]  FilterDenConstantOutMax=[]  PCopyOutDataTypeStr=Inherit: Inherit via back propagation  PCopyOutMin=[]  PCopyOutMax=[]  NCopyOutDataTypeStr=Inherit: Inherit via back propagation  NCopyOutMin=[]  NCopyOutMax=[]  IntegratorContinuousStateAttributes=''  IntegratorStateMustResolveToSignalObject=off  IntegratorRTWStateStorageClass=Auto  FilterContinuousStateAttributes=''  FilterStateMustResolveToSignalObject=off  FilterRTWStateStorageClass=Auto  ParallelPVariant=InternalParameters  IdealPVariant=Disabled  IVariant=InternalParameters  DVariant=Disabled  IntegratorVariant=Discrete  SatVariant=Disabled  AWVariant=Passthrough  PCopyVariant=Disabled  TRVariant=Disabled  FdbkBlocksVariant=Forward  IdealPFdbkVariant=Disabled  SatFdbkVariant=Disabled  DerivativeFilterVariant=Disabled  NVariant=Disabled  NCopyVariant=Disabled_SignalSpec  FilterICVariant=Disabled  IntegratorICVariant=InternalICs  ExternalResetVariant=Disabled  TRSumVariant=Passthrough  SumFdbkVariant=Disabled  SumVariant=Sum_PI  TsampFilterVariant=InternalTs  TsampNgainVariant=Passthrough  TsampIntegralVariant=Passthrough  ExternalSaturationOutDataTypeStr=Inherit: Same as second input
  z_motor_command : Outport
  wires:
  z_pos/1 -> Discrete D Controller/1
  z_error/1 -> Discrete PI Controller/1
  Discrete PI Controller/1 -> Add/1
  Discrete D Controller/1 -> Add/2
  Add/1 -> z_motor_command/1

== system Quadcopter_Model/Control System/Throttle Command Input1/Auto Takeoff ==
  height_controlled_o : Constant  Value=0.45  SampleTime=Tc
  z_command : Outport
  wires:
  height_controlled_o/1 -> z_command/1

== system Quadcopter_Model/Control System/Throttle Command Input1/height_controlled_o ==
  height_controlled_o : Constant  Value=height_controlled_o  SampleTime=Tc
  z_command : Outport
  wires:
  height_controlled_o/1 -> z_command/1

== matlab function Quadcopter_Model/Actuation/Aeb














 ==
function euler_rates = angular_body_earth_conversion(B_omega, euler_angles)

phi = euler_angles(1);
theta = euler_angles(2);

Aeb = [1,  sin(phi)*tan(theta), cos(phi)*tan(theta); ...
       0,      cos(phi)       ,        -sin(phi)   ; ...
       0,  sin(phi)/cos(theta), cos(phi)/cos(theta)];

   
euler_rates = Aeb * B_omega;

== matlab function Quadcopter_Model/Actuation/Lbe

















 ==
function [B_Fg, B_g]  = linear_earth_body_conversion(E_Fg, euler_angles, m)

phi = euler_angles(1);
theta = euler_angles(2);
psi = euler_angles(3);

Lbe = [             cos(theta)*cos(psi)              ,          cos(theta)*sin(psi)                  ,     -sin(theta)    ; ...
       sin(phi)*sin(theta)*cos(psi)-cos(phi)*sin(psi), sin(phi)*sin(theta)*sin(psi)+cos(phi)*cos(psi), sin(phi)*cos(theta); ...
       cos(phi)*sin(theta)*cos(psi)+sin(phi)*sin(psi), cos(phi)*sin(theta)*sin(psi)-sin(phi)*cos(psi), cos(phi)*cos(theta)];

B_Fg = Lbe * E_Fg;

B_g = B_Fg/m;

== matlab function Quadcopter_Model/     Sensors   /IMU





/






 ==
function [accelReading,gyroReading] = idealIMU(B_vo_dot, B_vo, B_Omega, B_g, g, r_oc)
%#codegen

a = B_vo_dot + cross(B_Omega,B_vo); % body frame acceleration 

accelReading = (a - B_g)/g ; % accelerometer reading (ideal)

gyroReading = B_Omega ; % gyroscope reading (ideal) 

end

== matlab function Quadcopter_Model/     Sensors   /Lbe





 ==
function B_vo  = linear_earth_body_conversion(E_vo, euler_angles)

phi = euler_angles(1);
theta = euler_angles(2);
psi = euler_angles(3);

Leb = [cos(theta)*cos(psi), sin(phi)*sin(theta)*cos(psi)-cos(phi)*sin(psi), cos(phi)*sin(theta)*cos(psi)+sin(phi)*sin(psi); ...
       cos(theta)*sin(psi), sin(phi)*sin(theta)*sin(psi)+cos(phi)*cos(psi), cos(phi)*sin(theta)*sin(psi)-sin(phi)*cos(psi); ...
           -sin(theta)    ,                sin(phi)*cos(theta)            ,                 cos(phi)*cos(theta)           ];

B_vo = Leb^-1 * E_vo;

== matlab function Quadcopter_Model/     Sensors   /Aeb









 ==
function euler_rates_IMU = angular_body_earth_conversion(gyro_reading, euler_angles_filtered)

phi = euler_angles_filtered(1);
theta = euler_angles_filtered(2);

Aeb = [1, sin(phi)*tan(theta), cos(phi)*tan(theta); ...
       0,     cos(phi)       ,        -sin(phi)   ; ...
       0,  sin(phi)/cos(theta), cos(phi)/cos(theta)];

   
euler_rates_IMU = Aeb * gyro_reading;

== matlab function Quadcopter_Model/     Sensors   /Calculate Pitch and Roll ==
function [accel_pitch, accel_roll] = getPitchAndRoll(accel_reading)

x_accel = accel_reading(1);
y_accel = accel_reading(2);
z_accel = accel_reading(3);

accel_pitch = atan(x_accel/sqrt(y_accel^2 + z_accel^2));
accel_roll = atan( -y_accel/( sqrt(z_accel^2 + x_accel^2))  );

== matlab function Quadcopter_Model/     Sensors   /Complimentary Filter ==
function euler_angles_IMU   = complimentaryFilter(accel_pitch, accel_roll, euler_rates_gyro, prev_euler_angles)

k_gyro = 0.99; 
k_accel = 1-k_gyro; 

Ts = 0.005; % 5 milliseconds

prev_phi = prev_euler_angles(1);
prev_theta = prev_euler_angles(2);

prev_phi_dot = euler_rates_gyro(1);
prev_theta_dot = euler_rates_gyro(2);

integrated_phi_gyro = Ts * prev_phi_dot + prev_phi;
integrated_theta_gyro = Ts * prev_theta_dot + prev_theta;

phi = k_gyro * integrated_phi_gyro + k_accel * accel_roll;
theta = k_gyro * integrated_theta_gyro + k_accel * accel_pitch;

euler_angles_IMU = [phi; theta];

== matlab function Quadcopter_Model/Actuation/Gravity

 ==
function E_Fg = gravity(m, g)

E_Fg = [0; 0; m*g];

== matlab function Quadcopter_Model/Actuation/Lbe





 ==
function E_ro  = linear_body_earth_conversion(B_vo, euler_angles)

euler_rates = zeros(3,1);
E_ro = zeros(3,1);

phi = euler_angles(1);
theta = euler_angles(2);
psi = euler_angles(3);

Leb = [cos(theta)*cos(psi), sin(phi)*sin(theta)*cos(psi)-cos(phi)*sin(psi), cos(phi)*sin(theta)*cos(psi)+sin(phi)*sin(psi); ...
       cos(theta)*sin(psi), sin(phi)*sin(theta)*sin(psi)+cos(phi)*cos(psi), cos(phi)*sin(theta)*sin(psi)-sin(phi)*cos(psi); ...
           -sin(theta)    ,                sin(phi)*cos(theta)            ,                 cos(phi)*cos(theta)           ];

E_ro = Leb * B_vo;

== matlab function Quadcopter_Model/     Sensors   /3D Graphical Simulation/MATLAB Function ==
function y = eigenaxis_ucart(u)


if abs(u(1))< 0.0001
    u(1) = 0.0001;
end

if abs(u(2))< 0.0001
    u(2) = 0.0001;
end

if abs(u(3))< 0.0001
    u(3) = 0.0001;
end

u = [ -u(1); -u(2); u(3) ];% [Pitch, Yaw, Roll] 

C11 = cos(u(2))*cos(u(3));
C12 = cos(u(2))*sin(u(3));
C13 = -sin(u(2));
C21 = sin(u(1))*sin(u(2))*cos(u(3))-cos(u(1))*sin(u(3));
C22 = sin(u(1))*sin(u(2))*sin(u(3))+cos(u(1))*cos(u(3));
C23 = sin(u(1))*cos(u(2));
C31 = cos(u(1))*sin(u(2))*cos(u(3))+sin(u(1))*sin(u(3));
C32 = cos(u(1))*sin(u(2))*sin(u(3))-sin(u(1))*cos(u(3));
C33 = cos(u(1))*cos(u(2));
    
theta = acos(0.5*(C11+C22+C33-1));

e = [C23-C32; C31-C13; C12-C21]/(2*sin(theta));
    
y = [e; theta];

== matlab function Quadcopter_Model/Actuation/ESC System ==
function Vb_eff   = ESC(P, Pmin, Pmax, Vb)

P1 = P(1);
P2 = P(2);
P3 = P(3);
P4 = P(4);

% Define u_Pi for each of the rotors, limiting it to be greater than 0
u_P0 = (P1 - Pmin) / (Pmax - Pmin);
u_P1 = (P2 - Pmin) / (Pmax - Pmin);
u_P2 = (P3 - Pmin) / (Pmax - Pmin);
u_P3 = (P4 - Pmin) / (Pmax - Pmin);


% Determine the effective battery voltage from each ESC
Vb_eff_0 = u_P0 * Vb;
Vb_eff_1 = u_P1 * Vb;
Vb_eff_2 = u_P2 * Vb;
Vb_eff_3 = u_P3 * Vb;
    
Vb_eff = [Vb_eff_0, Vb_eff_1, Vb_eff_2, Vb_eff_3];

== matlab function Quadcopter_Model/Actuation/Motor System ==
function w_dot = motor(Vb_eff, w, Rm, Kv, Kq, Kd, If, Jreq)

% Define each motors effective battery voltage
Vb_eff_0 = Vb_eff(1);
Vb_eff_1 = Vb_eff(2);
Vb_eff_2 = Vb_eff(3);
Vb_eff_3 = Vb_eff(4);

% Determine the angular velocity of each rotor from feedback
w_0 = w(1);
w_1 = w(2);
w_2 = w(3);
w_3 = w(4);

% Determine angular acceleration of each rotor
w_0_dot = 1/(Jreq*Rm*Kq) * Vb_eff_0 - 1/(Jreq*Rm*Kq*Kv) * w_0 - 1/(Jreq*Kq)*If - (Kd/Jreq) * w_0^2;
w_1_dot = 1/(Jreq*Rm*Kq) * Vb_eff_1 - 1/(Jreq*Rm*Kq*Kv) * w_1 - 1/(Jreq*Kq)*If - (Kd/Jreq) * w_1^2;
w_2_dot = 1/(Jreq*Rm*Kq) * Vb_eff_2 - 1/(Jreq*Rm*Kq*Kv) * w_2 - 1/(Jreq*Kq)*If - (Kd/Jreq) * w_2^2;
w_3_dot = 1/(Jreq*Rm*Kq) * Vb_eff_3 - 1/(Jreq*Rm*Kq*Kv) * w_3 - 1/(Jreq*Kq)*If - (Kd/Jreq) * w_3^2;

w_dot = [w_0_dot, w_1_dot, w_2_dot, w_3_dot];

== matlab function Quadcopter_Model/Actuation/Rotor System







 ==
function [B_omega_dot, B_vo_dot]= rotor(w_dot, w, B_Fg, B_omega, B_vo, m, Kt, Kd, rhx, rhy, rhz, Jreq, Jxx, Jyy, Jzz, r_oc, Kh, delta_T)

% Create J vector
J = [Jxx,  0 ,  0 ; ...
      0 , Jyy,  0 ; ...
      0 ,  0 , Jzz;];
  
r_oc_X = [0, -r_oc(3), r_oc(2); r_oc(3), 0, -r_oc(1); -r_oc(2), r_oc(1), 0];

% Create r_hi vector
rh_0 = [-rhx; rhy; -rhz];
rh_1 = [rhx; rhy; -rhz];
rh_2 = [-rhx; -rhy; -rhz];
rh_3 = [rhx; -rhy; -rhz];

% Calculate rotor hub velocity
vh_0 = B_vo + cross(B_omega,rh_0);
vh_1 = B_vo + cross(B_omega,rh_1); 
vh_2 = B_vo + cross(B_omega,rh_2); 
vh_3 = B_vo + cross(B_omega,rh_3); 

% Define 3x3 Identity Matrix
I = eye(3);

% Create gamma vectors
gamma_Ti = [0; 0; -1];
gamma_omega_03 = [0; 0; 1];  %Rotors 0 and 3 use this gamma_omega vector
gamma_omega_12 = [0; 0; -1]; %Rotors 1 and 2 use this gamma_omega vector
gamma_Hi = [ 1 0 0 ; 0 1 0 ; 0 0 0 ];

% Define angular velocities for each rotor
w_0 = w(1);
w_1 = w(2);
w_2 = w(3);
w_3 = w(4);

% Define angular acceleration for each rotor
w_0_dot = w_dot(1);
w_1_dot = w_dot(2);
w_2_dot = w_dot(3);
w_3_dot = w_dot(4);

% Define the thrust force
T_0 = (Kt * w_0 * w_0 + delta_T * vh_0 * w_0) * gamma_Ti; 
T_1 = (Kt * w_1 * w_1 + delta_T * vh_1 * w_1) * gamma_Ti;
T_2 = (Kt * w_2 * w_2 + delta_T * vh_2 * w_2) * gamma_Ti;
T_3 = (Kt * w_3 * w_3 + delta_T * vh_3 * w_3) * gamma_Ti;

% Define the in plane drag force
H_0 = -Kh * w_0 * gamma_Hi * vh_0;
H_1 = -Kh * w_1 * gamma_Hi * vh_1;
H_2 = -Kh * w_2 * gamma_Hi * vh_2;
H_3 = -Kh * w_3 * gamma_Hi * vh_3;

% Define the rotor force in the z-direction from each rotor
B_Fr_0 = T_0 + H_0;
B_Fr_1 = T_1 + H_1;
B_Fr_2 = T_2 + H_2;
B_Fr_3 = T_3 + H_3;

% Sum up the rotor forces in the z-direction from each vector to get the
% total body force in the z-direction
B_Fr = B_Fr_0 + B_Fr_1 + B_Fr_2 + B_Fr_3;

% Define the in-plane drag and induced torque produced by each rotor
 B_Q_d0 = -1 * Kd * w_0 * w_0 * gamma_omega_03;
 B_Q_d1 = -1 * Kd * w_1 * w_1 * gamma_omega_12;
 B_Q_d2 = -1 * Kd * w_2 * w_2 * gamma_omega_12;
 B_Q_d3 = -1 * Kd * w_3 * w_3 * gamma_omega_03;

% Sum up the total in-plane drag and induced torque to get the total
% in-plane drag and induced torque on the body
B_Q_d = B_Q_d0 + B_Q_d1 + B_Q_d2 + B_Q_d3;

% Define the force lever arm torque created from the force produced by each
% rotor in the z-direction
B_Q_F0 = cross( rh_0, B_Fr_0 );
B_Q_F1 = cross( rh_1, B_Fr_1 );
B_Q_F2 = cross( rh_2, B_Fr_2 );
B_Q_F3 = cross( rh_3, B_Fr_3 );

B_Q_F = B_Q_F0 + B_Q_F1 + B_Q_F2 + B_Q_F3;

% Define the change in angular momentum torque produced by each rotor 
B_Q_L0 = -1 * Jreq * ( cross(B_omega, w_0 * gamma_omega_03) + w_0_dot * gamma_omega_03 );
B_Q_L1 = -1 * Jreq * ( cross(B_omega, w_1 * gamma_omega_12) + w_1_dot * gamma_omega_12 ); 
B_Q_L2 = -1 * Jreq * ( cross(B_omega, w_2 * gamma_omega_12) + w_2_dot * gamma_omega_12 ); 
B_Q_L3 = -1 * Jreq * ( cross(B_omega, w_3 * gamma_omega_03) + w_3_dot * gamma_omega_03 );

% Sum up the total change in angular momentum torque produced by each rotor
B_Q_L = B_Q_L0 + B_Q_L1 + B_Q_L2 + B_Q_L3;
    
% Define the total rotor system torque as the sum of the in-plane drag and
% induced torque, force lever arm torque, and change in angular momentum
% torques
B_Q = B_Q_d + B_Q_F + B_Q_L;

% Define the body forces in the z-direction from each vector to get the
% total body force in the z-direction
B_F = B_Fr + B_Fg; 

% Determine the dynamics of the system
M = [m * I , -m * r_oc_X; 
    zeros(3,3), J];

dynamics = M^-1*[B_F - m*cross(B_omega,B_vo) - m*cross(B_omega,cross(B_omega,r_oc)) ; ... 
          B_Q - cross(B_omega,J*B_omega) - cross(r_oc,B_F) ];

% Define the body frame angular velocities
B_vo_dot = dynamics(1:3);

% Define the body frame linear velocities
B_omega_dot = dynamics(4:6);
